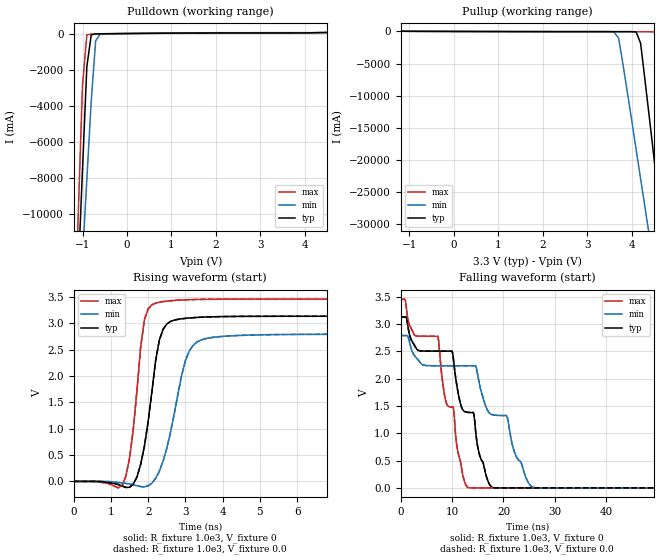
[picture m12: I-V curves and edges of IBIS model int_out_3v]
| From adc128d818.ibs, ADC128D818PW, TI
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[Model] int_out_3v
Model_type Output
Vmeas = 1.4V
Cref = 0.0pF
Rref = 1.0e3
Vref = 0.0V
C_comp   44.7pF   35.9pF   51.4pF
[Voltage Range]   3.3V   3.0V   3.6V
[Temperature Range]   25.0   125.0   -40.0
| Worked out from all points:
|   slope of the pulldown table from 0 to 0.495 V, typ, clamps not added: 43.7 ohm
|   slope of the pullup table from 0 to 0.495 V, typ, clamps not added: 55 ohm
|   rising waveform, R_fixture 1.0e3, V_fixture 0: 20-80 % time 369ps typ, 507ps min, 294ps max; typ from 0 V to 3.13 V
|   falling waveform, R_fixture 1.0e3, V_fixture 0: 20-80 % time 11ns typ, 8.03ns min, 3.82ns max; typ from 3.13 V to 0 V
|   rising waveform, R_fixture 1.0e3, V_fixture 0.0: 20-80 % time 369ps typ, 507ps min, 294ps max; typ from 0 V to 3.13 V
|   falling waveform, R_fixture 1.0e3, V_fixture 0.0: 20-80 % time 11ns typ, 8.03ns min, 3.82ns max; typ from 3.13 V to 0 V
[Pullup]
-3.3V     87.68mA    70.17mA    101.7mA
3.6V      -31.43mA   -75.17mA   -43.09mA
3.709V    -31.53mA   -1.026A    -43.25mA
4.105V    -88.97mA   -18.48A    -43.77mA
4.204V    -1.847A    -22.98A    -43.89mA
4.303V    -7.612A    -27.46A    -44.2mA
4.402V    -13.5A     -31.92A    -46.49mA
4.501V    -19.46A    -36.38A    -63.06mA
4.6V      -25.42A    -40.83A    -817.2mA
4.709V    -31.95A    -45.71A    -8.617A
5.006V    -49.68A    -58.99A    -31.29A
6.6V      -143.8A    -129.7A    -151.5A
[Pulldown]
-3.3V     -143.8A    -115.1A    -176.2A
-1.201V   -19.45A    -21.47A    -17.9A
-1.102V   -13.48A    -16.96A    -10.35A
-1.003V   -7.599A    -12.48A    -2.924A
-904.2mV  -1.833A    -8.071A    -77.56mA
-805.2mV  -74.74mA   -3.742A    -30.47mA
-706.2mV  -21.09mA   -408.3mA   -23.61mA
-607.2mV  -15.13mA   -37.99mA   -20.15mA
4.392V    53.63mA    54.06mA    48.56mA
6.6V      130.9mA    101mA      155.8mA
[Rising Waveform]
R_fixture=1.0e3
V_fixture=0
V_fixture_min=0
V_fixture_max=0
0s        1.523nV    79.33nV    1.201nV
1.3ns     -86.26mV   -29.96mV   -77.63mV
1.6ns     -50.57mV   -64.63mV   984.6mV
1.8ns     325.5mV    -98.45mV   2.559V
2ns       1.136V     -84.58mV   3.272V
2.3ns     2.678V     190.9mV    3.399V
2.9ns     3.084V     2.013V     3.441V
3.4ns     3.113V     2.676V     3.452V
5.4ns     3.131V     2.784V     3.456V
99.95ns   3.133V     2.791V     3.457V
[Falling Waveform]
R_fixture=1.0e3
V_fixture=0
V_fixture_min=0
V_fixture_max=0
0s        3.133V     2.791V     3.457V
2.7ns     2.613V     2.422V     2.8V
7.3ns     2.505V     2.236V     2.756V
8.6ns     2.504V     2.236V     1.669V
10ns      2.503V     2.236V     1.477V
13.2ns    1.382V     2.236V     4.183mV
17.5ns    33.78mV    1.353V     74.23uV
20.6ns    110.7uV    1.323V     68.5uV
25.7ns    73.22uV    11.65mV    45.14uV
99.95ns   -11.83uV   5.962uV    6.251uV
[Rising Waveform]
R_fixture=1.0e3
V_fixture=0.0
V_fixture_min=0.0
V_fixture_max=0.0
0s        1.523nV    79.33nV    1.201nV
1.3ns     -86.26mV   -29.96mV   -77.63mV
1.6ns     -50.57mV   -64.63mV   984.6mV
1.8ns     325.5mV    -98.45mV   2.559V
2ns       1.136V     -84.58mV   3.272V
2.3ns     2.678V     190.9mV    3.399V
2.9ns     3.084V     2.013V     3.441V
3.4ns     3.113V     2.676V     3.452V
5.4ns     3.131V     2.784V     3.456V
99.95ns   3.133V     2.791V     3.457V
[Falling Waveform]
R_fixture=1.0e3
V_fixture=0.0
V_fixture_min=0.0
V_fixture_max=0.0
0s        3.133V     2.791V     3.457V
2.7ns     2.613V     2.422V     2.8V
7.3ns     2.505V     2.236V     2.756V
8.6ns     2.504V     2.236V     1.669V
10ns      2.503V     2.236V     1.477V
13.2ns    1.382V     2.236V     4.183mV
17.5ns    33.78mV    1.353V     74.23uV
20.6ns    110.7uV    1.323V     68.5uV
25.7ns    73.22uV    11.65mV    45.14uV
99.95ns   -11.83uV   5.962uV    6.251uV
[Ramp]
R_load = 1.0e3
dV/dt_r   1.87955E0/4E-10   1.674829E0/5E-10   2.074007E0/3E-10
dV/dt_f   1.879556E0/1.09E-8   1.674825E0/8E-9   2.074002E0/3.8E-9
